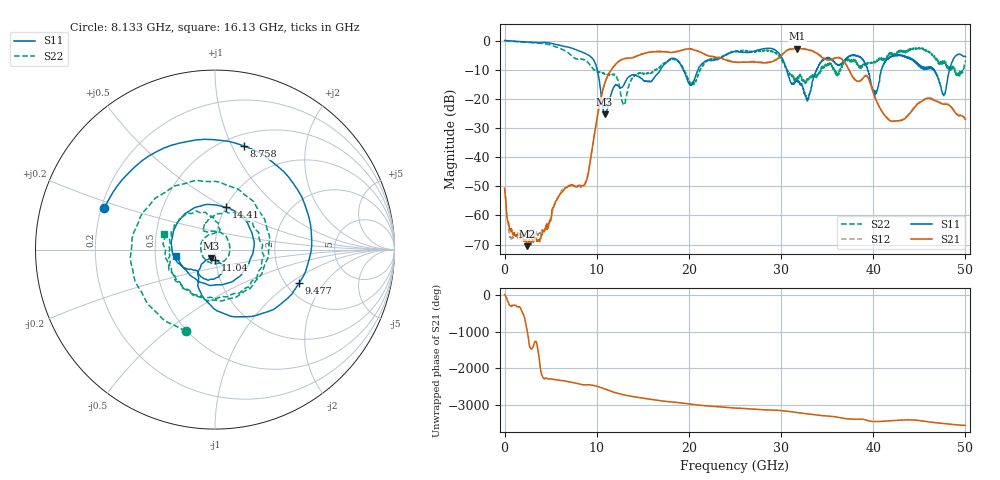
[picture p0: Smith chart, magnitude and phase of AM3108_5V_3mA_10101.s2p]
# Hz S DB R 50.0
!freq dBS11 angS11 dBS21 angS21 dBS12 angS12 dBS22 angS22
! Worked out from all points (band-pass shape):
!   1601 points, 10 MHz to 50 GHz, reference 50 ohm
!   highest |S21| = -2.77 dB at 31.78 GHz (marker M1); lowest = -70.6 dB at 2.447 GHz (marker M2)
!   |S21| within 3 dB of the highest: 14.05 GHz to 22.94 GHz (8.897 GHz wide, 48.1 % of centre); 29.85 GHz to 34.44 GHz (4.585 GHz wide, 14.3 % of centre)
!   lowest |S11| = -25.4 dB at 10.85 GHz (marker M3), VSWR 1.11, Z = 47.7 - j4.72 ohm
!   |S11| at or under -10 dB: 10.06 GHz to 16.92 GHz (6.86 GHz wide, 50.9 % of centre); 30.62 GHz to 33.84 GHz (3.229 GHz wide, 10 % of centre); 46.62 GHz to 48.28 GHz (1.666 GHz wide, 3.51 % of centre)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
!   |S22| runs from -22.2 to 0.0 dB; largest |S21 - S12| = 0.026
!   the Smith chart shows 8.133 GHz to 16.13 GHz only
!   S11 on the Smith chart (normalised r, x): 8.133 GHz: 0.21, +0.17; 8.758 GHz: 0.62, +1.11; 9.477 GHz: 2.35, -1.18; 11.04 GHz: 0.99, -0.12; 14.41 GHz: 1.00, +0.50; 16.13 GHz: 0.64, -0.05
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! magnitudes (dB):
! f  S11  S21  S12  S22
! 10 MHz  0.0  -50.7  -50.6  0.0
! 697.4 MHz  -0.1  -65.0  -67.6  -0.2
! 2.447 GHz  -0.5  -70.6  -68.2  -0.6
! 8.133 GHz  -3.6  -49.7  -50.0  -6.3
! 8.352 GHz  -3.9  -49.9  -50.2  -6.3
! 8.758 GHz  -4.4  -49.2  -48.7  -6.8
! 9.477 GHz  -5.9  -37.9  -37.8  -9.2
! 10.85 GHz  -25.4  -14.9  -14.9  -11.3
! 11.04 GHz  -24.7  -13.2  -13.2  -11.6
! 12.94 GHz  -15.4  -6.3  -6.1  -22.0
! 14.41 GHz  -12.3  -5.2  -5.1  -11.6
! 16.13 GHz  -13.1  -3.9  -3.8  -10.5
! 16.69 GHz  -11.0  -3.9  -3.6  -9.7
! 20.41 GHz  -14.5  -3.1  -2.9  -15.4
! 25 GHz  -3.8  -7.4  -7.3  -3.8
! 31.78 GHz  -14.2  -2.8  -2.7  -13.6
! 33.35 GHz  -15.5  -3.6  -3.4  -12.7
! 38 GHz  -5.0  -13.5  -13.3  -6.6
! 40.22 GHz  -18.7  -19.8  -19.6  -7.6
! 41.69 GHz  -6.0  -27.2  -26.9  -5.2
! 47.66 GHz  -18.9  -21.8  -21.5  -7.7
! 50 GHz  -5.5  -27.1  -26.5  -6.9
